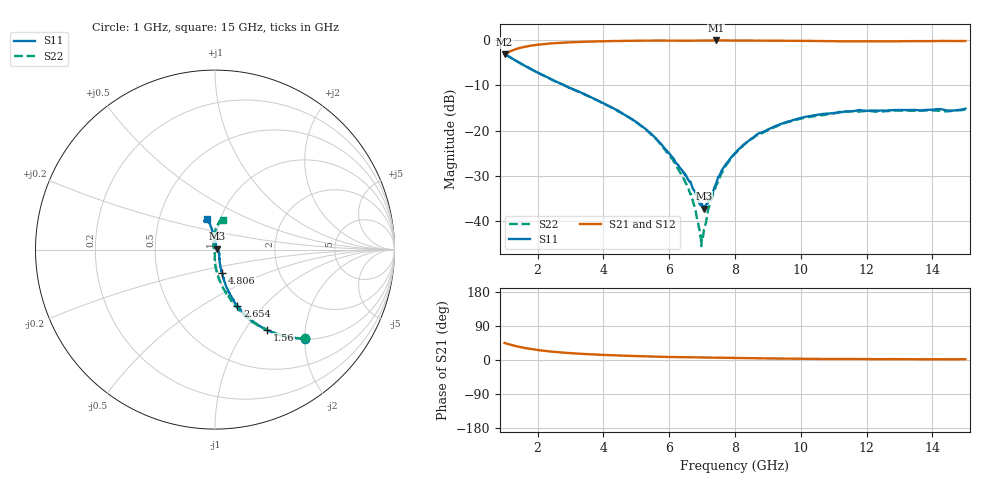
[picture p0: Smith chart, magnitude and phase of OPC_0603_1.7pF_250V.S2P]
! FILE NAME
! DATE 08/20/2012  15:12
! CORRECTED  DATA
# GHz  S  MA  R  50.00
!  FREQ  S11M  S11A  S21M  S21A  S12M  S12A  S22M  S22A
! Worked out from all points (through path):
!   1601 points, 1 GHz to 15 GHz, reference 50 ohm
!   highest |S21| = -0.06 dB at 7.423 GHz (marker M1); lowest = -3.1 dB at 1 GHz (marker M2)
!   group delay of S21, straight-line fit = 5.3 ps
!   lowest |S11| = -37.3 dB at 7.055 GHz (marker M3), VSWR 1.03, Z = 51.3 + j0.504 ohm
!   |S11| at or under -10 dB: 2.822 GHz to end of sweep
!   |S22| runs from -45.6 to -3.1 dB; largest |S21 - S12| = 0.0079
!   S11 on the Smith chart (normalised r, x): 1 GHz: 1.02, -2.00; 1.56 GHz: 1.02, -1.28; 2.654 GHz: 1.03, -0.73; 4.806 GHz: 1.04, -0.28; 15 GHz: 0.86, +0.30
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1  0.704 -44.7  0.7015 44.9  0.7016 44.9  0.7036 -44.7
1.56  0.5341 -56.9  0.837 32.5  0.8372 32.5  0.5337 -57.1
2.65375  0.3377 -68.2  0.9329 20.4  0.9323 20.4  0.336 -69.7
3.33625  0.2616 -71.6  0.9583 16.3  0.9581 16.3  0.2601 -75.0
4.80625  0.1377 -73.3  0.9848 10.9  0.9842 10.9  0.1373 -84.3
5.6725  0.07645 -70.2  0.9906 8.7  0.9906 8.7  0.07537 -90.4
6.10125  0.05055 -60.8  0.9884 7.8  0.988 7.8  0.048 -91.6
6.495  0.03266 -45.2  0.987 7.3  0.9864 7.4  0.02673 -91.6
6.7225  0.02257 -31.1  0.9889 7.2  0.9886 7.2  0.01639 -101.4
6.95  0.01524 -2.0  0.9907 6.8  0.9902 6.8  0.006758 -153.8
7.0025  0.01508 7.2  0.9911 6.7  0.9909 6.8  0.006007 -178.2
7.055  0.01372 21.0  0.9917 6.6  0.9917 6.7  0.007975 151.8
7.23  0.0176 54.2  0.992 6.4  0.992 6.4  0.01509 114.8
7.4225  0.02589 77.9  0.9933 6.1  0.9923 6.1  0.02433 107.2
7.65  0.03884 85.2  0.9927 5.8  0.9922 5.8  0.03707 103.2
8  0.05629 91.7  0.9922 5.3  0.9915 5.3  0.05551 98.2
8.7175  0.093 96.5  0.9898 4.5  0.9895 4.5  0.0901 90.7
9.51375  0.1225 99.6  0.9858 3.7  0.9858 3.7  0.1211 86.9
10.33625  0.146 101.3  0.9812 3.0  0.9805 3.0  0.1428 82.5
11.2375  0.1597 104.6  0.9728 2.7  0.9726 2.7  0.1627 79.9
12.6725  0.1672 108.8  0.9701 2.4  0.9703 2.4  0.1646 77.0
15  0.1749 105.5  0.9804 2.2  0.9804 2.2  0.1714 75.0
